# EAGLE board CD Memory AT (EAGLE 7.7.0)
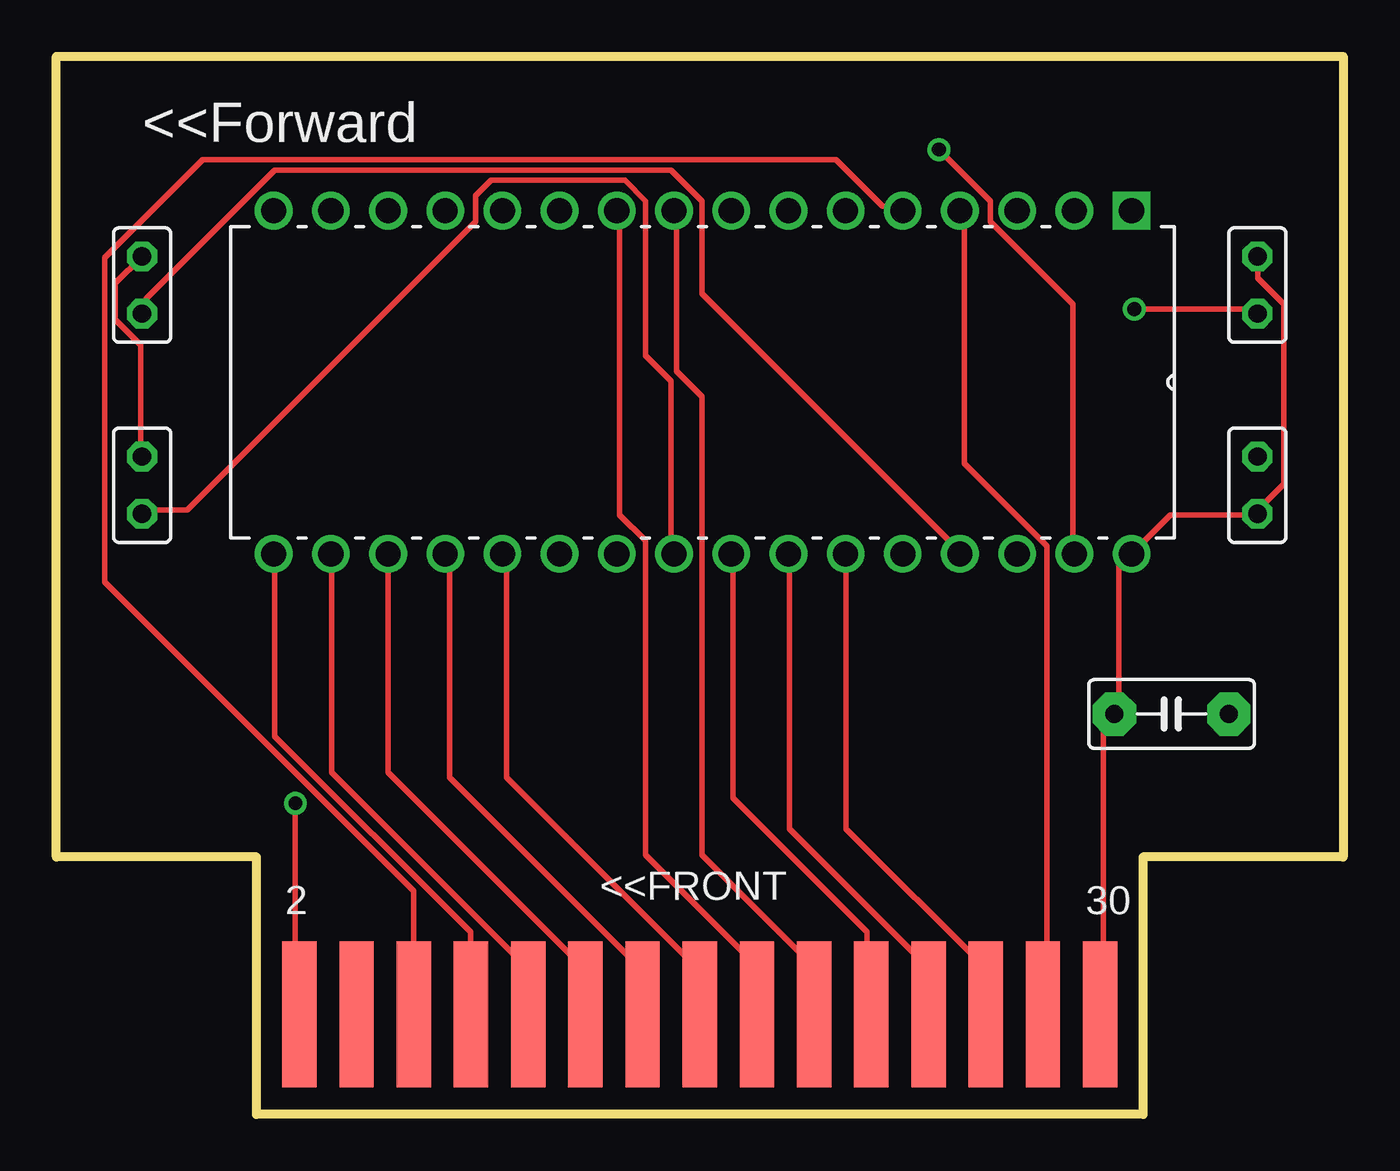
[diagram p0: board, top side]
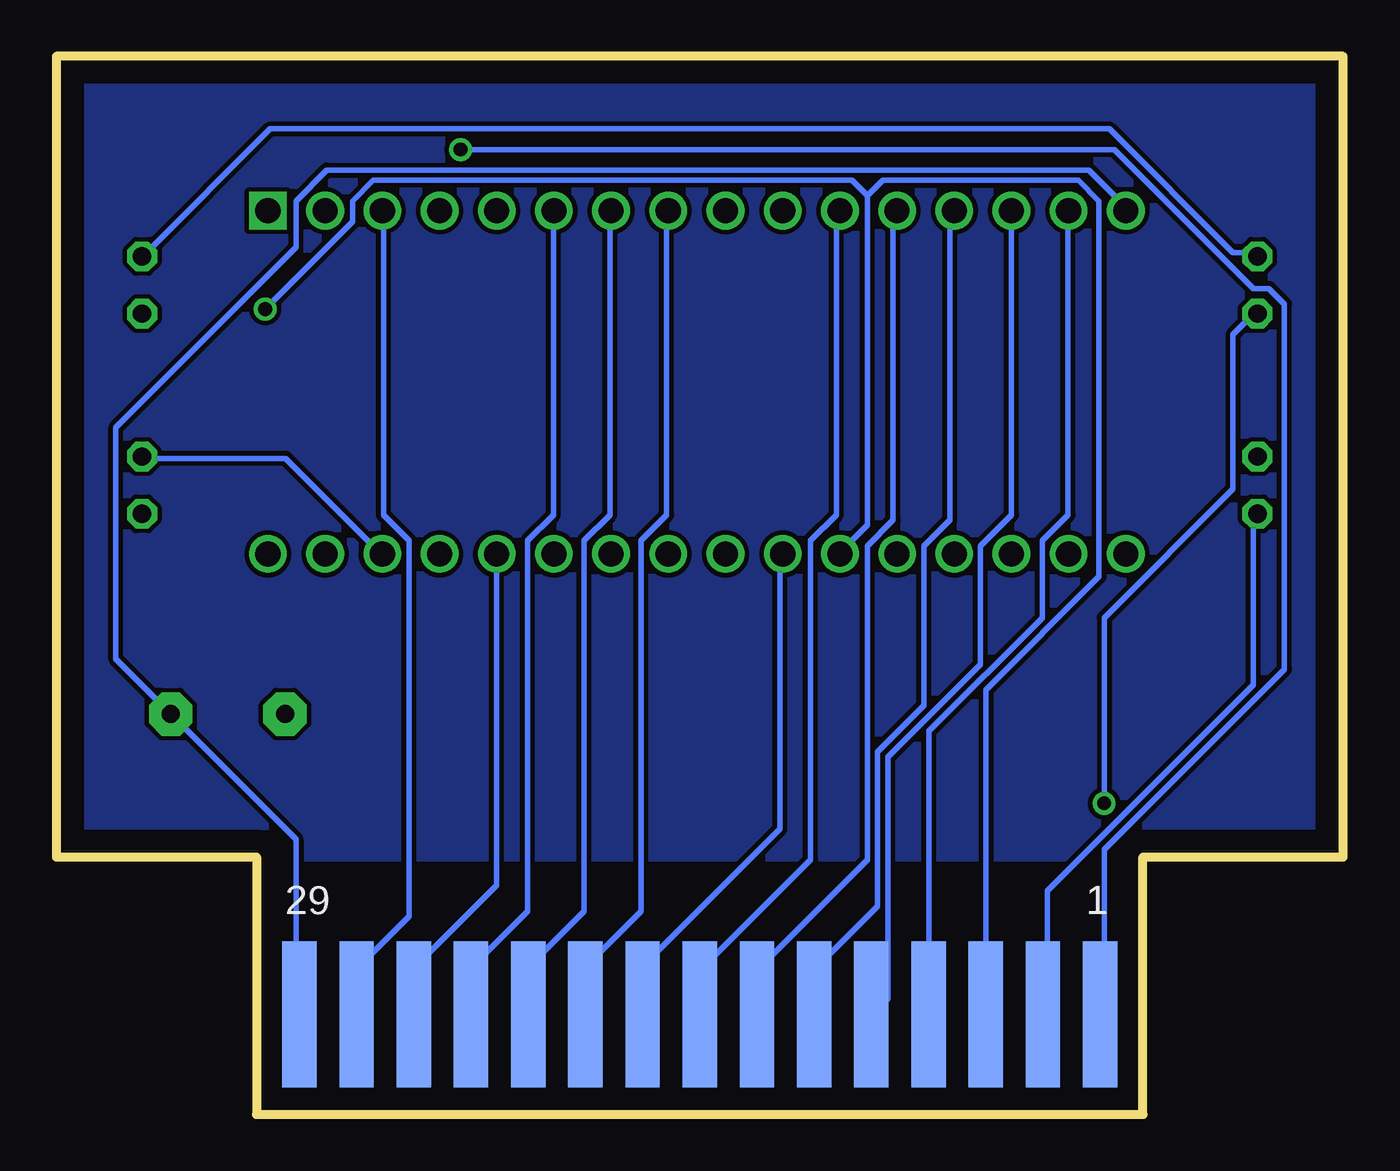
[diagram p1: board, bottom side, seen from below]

Size 57.15 x 46.99 mm. Coordinates in mm from the lower left corner, seen from the top.
Outline: 8.89,11.43 0,11.43 0,46.99 57.15,46.99 57.15,11.43 48.26,11.43 48.26,0 8.89,0 8.89,11.43
Copper layers (1*16): Top 0.035mm / dielectric 1.5mm / Bottom 0.035mm
Design rules "default": minimum track width 10mil, minimum drill 24mil, track to track 8mil, track to pad 8mil, pad to pad 8mil, via to via 8mil, smd to smd 8mil, copper to edge 40mil, drill to drill 8mil, minimum pad ring 10mil, minimum via ring 8mil, stop-mask expansion 4mil, vias tented up to drill 0mil, thermal gap 10mil

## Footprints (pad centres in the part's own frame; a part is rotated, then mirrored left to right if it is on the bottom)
C050-030X075 = drill 0.813 pad 1.93 octagon: 1 -2.54,0; 2 2.54,0
DIP254P1524X393-32 = drill 1.118 pad 1.676 square: 1 -15.24,38.1 | drill 1.118 pad 1.676: 2 -15.24,35.56; 3 -15.24,33.02; 4 -15.24,30.48; 5 -15.24,27.94; 6 -15.24,25.4; 7 -15.24,22.86; 8 -15.24,20.32; 9 -15.24,17.78; 10 -15.24,15.24; 11 -15.24,12.7; 12 -15.24,10.16; 13 -15.24,7.62; 14 -15.24,5.08; 15 -15.24,2.54; 16 -15.24,0; 17 0,0; 18 0,2.54; 19 0,5.08; 20 0,7.62; 21 0,10.16; 22 0,12.7; 23 0,15.24; 24 0,17.78; 25 0,20.32; 26 0,22.86; 27 0,25.4; 28 0,27.94; 29 0,30.48; 30 0,33.02; 31 0,35.56; 32 0,38.1
V526-0 = drill 0.813 octagon: 1 -1.27,0; 2 1.27,0
J5CARD_NO_OUTLINE = smd 1.524 x 6.477 bottom: 1 -18.415,-5.715; 3 -15.875,-5.715; 5 -13.335,-5.715; 7 -10.795,-5.715; 9 -8.255,-5.715; 11 -5.715,-5.715; 13 -3.175,-5.715; 15 -0.635,-5.715; 17 1.905,-5.715; 19 4.445,-5.715; 21 6.985,-5.715; 23 9.525,-5.715; 25 12.065,-5.715; 27 14.605,-5.715; 29 17.145,-5.715 | smd 1.524 x 6.477: 2 -18.415,-5.715; 4 -15.875,-5.715; 6 -13.335,-5.715; 8 -10.795,-5.715; 10 -8.255,-5.715; 12 -5.715,-5.715; 14 -3.175,-5.715; 16 -0.635,-5.715; 18 1.905,-5.715; 20 4.445,-5.715; 22 6.985,-5.715; 24 9.525,-5.715; 26 12.065,-5.715; 28 14.605,-5.715; 30 17.145,-5.715

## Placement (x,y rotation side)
C1  0.1uf  [C050-030X075]  49.53,17.78 180 top
IC1  AS6C1008-55PCN  [DIP254P1524X393-32]  9.65,24.89 270 top
R1  10K  [V526-0]  53.34,27.94 270 top
R2  10k  [V526-0]  3.81,36.83 90 top
R3  10K  [V526-0]  3.81,27.94 90 top
R4  10K  [V526-0]  53.34,36.83 90 top
U$1  MEM_CARD_NO_OUTLINE  [J5CARD_NO_OUTLINE]  29.21,10.16 0 top

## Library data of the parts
C1 R1-R4 = rcl
IC1 = SamacSys_Parts; DESCRIPTION: CMOS SRAM; HEIGHT: mm; MANUFACTURER_NAME: Alliance Memory; MANUFACTURER_PART_NUMBER: AS6C1008-55PCN; MOUSER_PART_NUMBER: 913-AS6C1008-55PCN; MOUSER_PRICE-STOCK: https://www.mouser.co.uk/ProductDetail/Alliance-Memory/AS6C1008-55PCN?qs=E5c5%252Bmu3i39qb4Qta5D2qg%3D%3D
U$1 = ADAM

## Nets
A0: IC1.12 U$1.13
A1: IC1.11 U$1.15
A2: IC1.10 U$1.18
A3: IC1.9 U$1.20
A4: IC1.8 U$1.19
A5: IC1.7 U$1.21
A6: IC1.6 U$1.23
A7: IC1.5 U$1.6
A8: IC1.27 U$1.26
A9: IC1.26 U$1.24
A10: IC1.23 U$1.17
A11: IC1.25 U$1.22
A12: IC1.4 U$1.28
A13: IC1.28 U$1.25
A14: IC1.3 U$1.27
A15: IC1.31 U$1.1
CS: IC1.22 R4.1 U$1.5
D0: IC1.13 U$1.11
D1: IC1.14 U$1.9
D2: IC1.15 U$1.7
D3: IC1.17 U$1.8
D4: IC1.18 U$1.10
D5: IC1.19 U$1.12
D6: IC1.20 U$1.14
D7: IC1.21 U$1.16
N$1: IC1.30 R1.1
OE: IC1.24 R3.1 U$1.3
VCC: C1.2 IC1.32 R1.2 R2.2 R3.2 R4.2 U$1.30
VSS: C1.1 IC1.16 U$1.29
WR: IC1.29 R2.1 U$1.2

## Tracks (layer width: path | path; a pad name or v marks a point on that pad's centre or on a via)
A0
  Bottom 0.254: IC1.12 19.99,40.11 19.99,26.39 21.13,25.25 21.13,11.3 25.93,6.5 25.93,4.45 U$1.13
A1
  Bottom 0.254: IC1.11 22.5,40.11 22.5,26.62 23.65,25.48 23.65,11.3 28.45,6.5 28.45,4.45 U$1.15
A2
  Top 0.254: IC1.10 25.02,40.11 25.02,26.62 26.16,25.48 26.16,11.53 30.96,6.73 30.96,4.45 U$1.18
A3
  Top 0.254: IC1.9 27.53,40.11 27.53,33.02 28.68,31.88 28.68,11.53 33.48,6.73 33.48,4.45 U$1.20
A4
  Bottom 0.254: IC1.8 30.05,40.11 30.05,26.62 31.19,25.48 31.19,9.02 33.48,6.73 33.48,4.45 U$1.19
A5
  Bottom 0.254: IC1.7 32.56,40.11 32.56,26.62 33.71,25.48 33.71,9.02 35.99,6.73 35.99,4.45 U$1.21
A6
  Bottom 0.254: U$1.23 38.73,6.5 36.22,9.02 36.22,25.48 35.08,26.62 35.08,40.11 IC1.6
A7
  Top 0.254: U$1.6 15.88,9.93 2.16,23.65 2.16,38.05 6.5,42.39 34.62,42.39 36.68,40.33 37.59,40.33 IC1.5
A8
  Top 0.254: IC1.27 35.08,24.79 35.08,12.68 41.25,6.5 41.25,4.45 U$1.26
A9
  Top 0.254: U$1.24 38.73,6.5 32.56,12.68 32.56,24.79 IC1.26
A10
  Bottom 0.254: IC1.23 25.02,24.79 25.02,12.68 30.96,6.73 30.96,4.45 U$1.17
A11
  Top 0.254: IC1.25 30.05,24.79 30.05,14.05 35.99,8.1 35.99,4.45 U$1.22
A12
  Top 0.254: IC1.4 40.33,40.11 40.33,28.91 43.99,25.25 43.99,4.45 U$1.28
A13
  Bottom 0.254: IC1.28 37.59,10.16 41.25,6.5 41.25,4.45 U$1.25
A14
  Bottom 0.254: IC1.3 42.62,40.11 42.62,26.62 41.48,25.48 41.48,8.79 43.76,6.5 43.76,4.45 U$1.27
A15  (via drill 0.61)
  Top 0.254: v39.19,42.85 41.48,40.56 41.48,39.65 45.14,35.99 45.14,25.02 IC1.31
  Bottom 0.254: v39.19,42.85 10.16,42.85 3.99,36.68 3.3,36.68 2.62,35.99 2.62,19.76 10.62,11.76 10.62,4.45 U$1.1
CS  (via drill 0.61)
  Top 0.254: v47.88,35.76 53.14,35.76 R4.1
  Bottom 0.254: v47.88,35.76 43.99,39.65 43.99,40.56 43.08,41.48 21.82,41.48 21.13,40.79 | 21.13,40.79 21.13,26.16 22.28,25.02 IC1.22 | U$1.5 15.88,18.85 10.85,23.88 10.85,40.56 11.76,41.48 20.45,41.48 21.13,40.79
D0
  Bottom 0.254: IC1.13 17.48,40.11 17.48,26.39 18.62,25.25 18.62,18.16 20.68,16.1 20.68,9.25 23.42,6.5 23.42,4.45 U$1.11
D1
  Bottom 0.254: IC1.14 14.73,26.62 16.1,25.25 16.1,19.99 20.22,15.88 20.22,5.13 20.9,4.45 U$1.9
D2
  Bottom 0.254: IC1.15 12.22,40.11 12.22,26.62 13.36,25.48 13.36,22.05 18.39,17.02 18.39,4.45 U$1.7
D3
  Top 0.254: IC1.17 9.7,24.79 9.7,16.79 18.39,8.1 18.39,4.45 U$1.8
D4
  Top 0.254: IC1.18 12.22,24.79 12.22,15.19 20.9,6.5 20.9,4.45 U$1.10
D5
  Top 0.254: IC1.19 14.73,15.19 23.42,6.5 23.42,4.45 U$1.12
D6
  Top 0.254: IC1.20 17.48,24.79 17.48,14.96 25.93,6.5 25.93,4.45 U$1.14
D7
  Top 0.254: IC1.21 19.99,24.79 19.99,14.96 28.45,6.5 28.45,4.45 U$1.16
GND
  pour Bottom: 57.15,11.43 0,11.43 0,46.99 57.15,46.99
N$1
  Bottom 0.254: R1.1 53.14,29.13 46.96,29.13 42.85,25.02 IC1.30
OE
  Top 0.254: IC1.24 27.3,25.02 27.3,32.56 26.16,33.71 26.16,40.56 25.25,41.48 19.3,41.48 18.62,40.79 18.62,39.65 5.82,26.85 3.99,26.85 R3.1
  Bottom 0.254: R3.1 3.99,26.62 3.99,19.07 13.13,9.93 13.13,4.45 U$1.3
VCC
  Top 0.254: R2.2 2.62,36.91 2.62,35.31 3.76,34.16 3.76,29.36 R3.2 | R4.2 53.36,38.05 53.36,37.13 54.51,35.99 54.51,27.99 53.36,26.85 R1.2 53.14,26.62 49.48,26.62 IC1.32 47.19,24.33 47.19,17.93 C1.2 46.96,17.7 46.51,17.25 46.51,4.45 U$1.30
  Bottom 0.254: R2.2 3.99,38.28 4.9,38.28 10.39,43.76 47.65,43.76 53.14,38.28 R4.2
VSS
  Bottom 0.254: IC1.16 9.7,40.33 11.3,41.93 45.14,41.93 46.51,40.56 46.51,38.51 54.51,30.5 54.51,20.22 C1.1 46.51,12.22 46.51,4.45 U$1.29
WR  (via drill 0.61)
  Top 0.254: R2.1 3.99,35.76 3.99,36.22 9.7,41.93 27.3,41.93 28.68,40.56 28.68,36.45 40.11,25.02 IC1.29 | v10.62,13.82 10.62,4.45 U$1.2
  Bottom 0.254: v10.62,13.82 10.62,22.05 4.9,27.76 4.9,34.62 3.99,35.53 R2.1

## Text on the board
tNames: <<Forward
